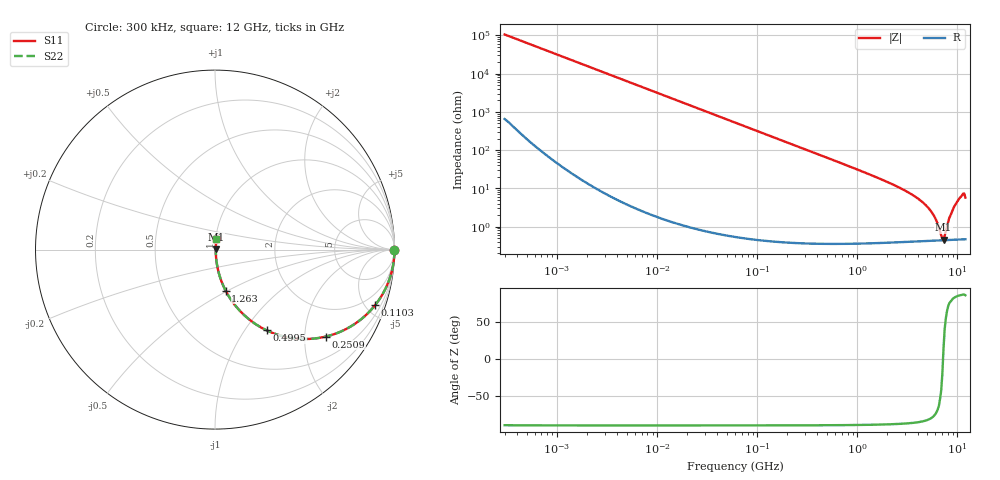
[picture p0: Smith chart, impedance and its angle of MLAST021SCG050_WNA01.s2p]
! MLAST021SCG050_WNA01  S-PARAMETER MODEL  ( General Type )
! Model Generated by TAIYO YUDEN Corporation (http://www.ty-top.com)
! Version 1.0
! TAIYO YUDEN Control No. 220901
! Copyright(c) 2022 TAIYO YUDEN CO.,LTD. All Rights Reserved.
! Product Description (link to TY-COMPAS)
! https://ds.yuden.co.jp/TYCOMPAS/or/detail?pn=MLAST021SCG050BWNA01&u=M
! Products Name : Multilayer Ceramic Capacitors
! Characteristics :
!  Capacitance : 5 pF , Rated Voltage : 25V , TCC : CG / C0G
!  Case Size : 0.25 x 0.125 / 0.0098 x 0.0049 [mm/inch] , Thickness : 0.125 / 0.0049 [mm/inch]
!  (Conditions: Temperature = 25 degC , DC Bias Current/Voltage = 0A / 0V)
! External Node Assignments :
!  1  o---| |---o  2
! GND o---------o GND
! Frequency Range : 0.3MHz  -  12000MHz  [ 401 STEP ]
# MHz S RI R 50
! Freq[MHz].  S11 Real  S11 Imag  S21 Real  S21 Imag  S12 Real  S12 Imag  S22 Real  S22 Imag
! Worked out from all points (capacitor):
!   401 points, 300 kHz to 12 GHz, reference 50 ohm
!   read as one part in series: C = 5 pF near 316.3 kHz
!   lowest |Z| = 455 mohm at 7.254 GHz (marker M1)
!   series resonance near 7.179 GHz, so ESL is about 98 pH
!   S11 on the Smith chart (normalised r, x): 300 kHz: open; 110.3 MHz: 1.01, -5.77; 250.9 MHz: 1.01, -2.53; 499.5 MHz: 1.01, -1.27; 1.263 GHz: 1.01, -0.49; 12 GHz: 1.01, +0.11
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0.3  1 -0.000942  6.7e-06 0.000942  6.7e-06 0.000942  1 -0.000942
1.769972  1 -0.00556  3.61e-05 0.00556  3.61e-05 0.00556  1 -0.00556
10.44266  0.9989 -0.0328  0.00109 0.0328  0.00109 0.0328  0.9989 -0.0328
60  0.9655 -0.182  0.0345 0.182  0.0345 0.182  0.9655 -0.182
110.3493  0.8923 -0.3092  0.1077 0.3092  0.1077 0.3092  0.8923 -0.3092
250.8588  0.616 -0.4849  0.384 0.4849  0.384 0.4849  0.616 -0.4849
353.9943  0.4461 -0.4951  0.5539 0.4951  0.5539 0.4951  0.4461 -0.4951
499.5319  0.2879 -0.45  0.7121 0.45  0.7121 0.45  0.2879 -0.45
783.7017  0.1409 -0.3436  0.8591 0.3436  0.8591 0.3436  0.1409 -0.3436
1262.535  0.0594 -0.229  0.9406 0.229  0.9406 0.229  0.0594 -0.229
2088.533  0.0227 -0.1359  0.9773 0.1359  0.9773 0.1359  0.0227 -0.1359
3454.93  0.00896 -0.0699  0.991 0.0699  0.991 0.0699  0.00896 -0.0699
4747.894  0.0056 -0.0374  0.9944 0.0374  0.9944 0.0374  0.0056 -0.0374
5715.274  0.0047 -0.0203  0.9953 0.0203  0.9953 0.0203  0.0047 -0.0203
6188.031  0.0045 -0.0132  0.9955 0.0132  0.9955 0.0132  0.0045 -0.0132
6879.757  0.0044 -0.00405  0.9956 0.00405  0.9956 0.00405  0.0044 -0.00405
7254.098  0.00441 0.00105  0.9956 -0.00105  0.9956 -0.00105  0.00441 0.00105
7448.838  0.00444 0.00364  0.9956 -0.00364  0.9956 -0.00364  0.00444 0.00364
8503.825  0.00485 0.0188  0.9952 -0.0188  0.9952 -0.0188  0.00485 0.0188
9454.42  0.00583 0.0357  0.9942 -0.0357  0.9942 -0.0357  0.00583 0.0357
11083.22  0.00877 0.0641  0.9912 -0.0641  0.9912 -0.0641  0.00877 0.0641
12000  0.00791 0.0567  0.9921 -0.0567  0.9921 -0.0567  0.00791 0.0567
